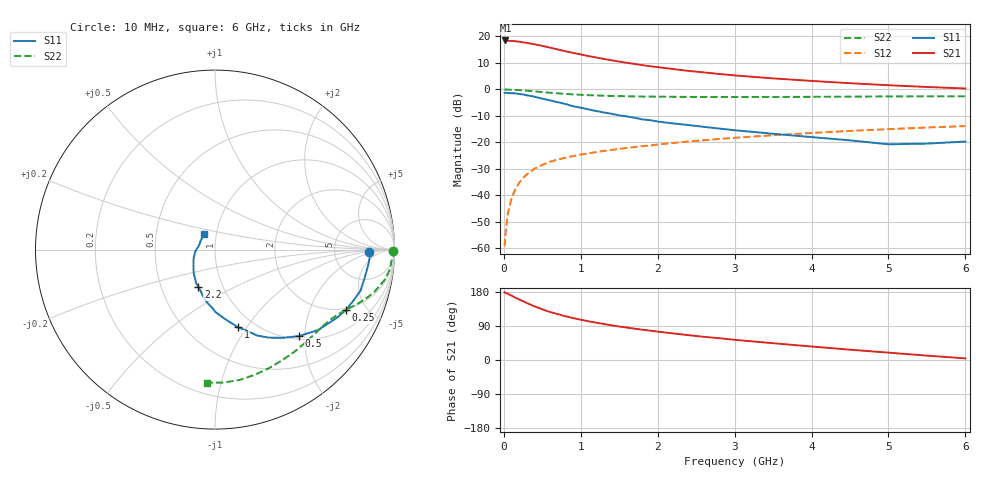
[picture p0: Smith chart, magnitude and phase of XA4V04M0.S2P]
! SIEMENS Discrete & RF Semiconductors
! BFY180
! Si NPN RF Bipolar Junction Transistor in MICRO-X
! VCE = 4 V  IC = 4 mA
! Common Emitter S-Parameters:  May  1997
# GHz  S  MA  R  50
!  f  S11  S21  S12  S22
! GHz  MAG  ANG  MAG  ANG  MAG  ANG  MAG  ANG
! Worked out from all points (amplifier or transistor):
!   36 points, 10 MHz to 6 GHz, reference 50 ohm
!   highest |S21| = 18.5 dB at 20 MHz (marker M1)
!   |S21| within 3 dB of that: start of sweep to 642.7 MHz
!   unconditionally stable (mu >= 1): 1.828 GHz to end of sweep
!   at 250 MHz: K = 0.21, MSG = 25.6 dB, |S12| = -33.4 dB
!   at 1.4 GHz: K = 0.89, MSG = 16.9 dB, |S12| = -22.8 dB
!   at 6 GHz: K = 1.07, MAG = 5.4 dB, |S12| = -13.8 dB
!   S11 on the Smith chart (normalised r, x): 10 MHz: 13, -1; 250 MHz: 1.89, -3.59; 500 MHz: 1.07, -1.87; 1 GHz: 0.84, -0.91; 2.2 GHz: 0.77, -0.34; 6 GHz: 0.87, +0.15
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0.01  0.8582 -0.9  8.31 178.4  0.0011 89.8  0.9896 -0.3
0.02  0.8644 -1.9  8.409 177.4  0.0018 89.6  0.9996 -0.8
0.05  0.8597 -5.0  8.265 174.8  0.0044 86.5  0.9913 -2.1
0.1  0.8488 -10.5  8.255 169.8  0.0089 84.9  0.984 -4.2
0.2  0.8211 -20.4  7.968 159.6  0.0174 79.2  0.9708 -8.1
0.25  0.8029 -24.9  7.744 155.1  0.0213 77.0  0.9603 -10.1
0.3  0.777 -29.4  7.583 150.2  0.025 73.0  0.9463 -11.6
0.4  0.7282 -38.0  7.108 141.5  0.032 69.9  0.9201 -14.7
0.5  0.6719 -45.8  6.645 133.7  0.0377 65.6  0.8916 -17.3
0.6  0.6204 -52.4  6.157 126.6  0.0432 63.4  0.8662 -19.4
0.8  0.5315 -64.1  5.254 115.4  0.0513 58.5  0.8242 -22.9
1  0.4518 -73.5  4.573 106.2  0.0589 56.2  0.7925 -25.8
1.1  0.4202 -77.3  4.268 102.3  0.0622 54.7  0.78 -27.1
1.2  0.3919 -81.6  4.013 98.4  0.0656 54.2  0.7707 -28.4
1.5  0.3239 -92.7  3.362 88.3  0.0754 52.0  0.7478 -32.3
1.7  0.2922 -99.6  3.032 82.6  0.0819 51.2  0.7381 -34.8
2.2  0.2284 -113.9  2.428 70.1  0.0977 48.3  0.7259 -41.5
3  0.1701 -134.4  1.841 53.3  0.1222 43.3  0.7211 -51.9
3.5  0.1455 -146.0  1.617 44.3  0.1365 40.1  0.721 -58.4
4.5  0.1094 -175.7  1.311 27.2  0.1648 32.9  0.7314 -71.9
5.5  0.0949 145.9  1.114 11.5  0.1912 25.1  0.7424 -86.2
6  0.1038 125.4  1.042 4.3  0.2033 20.9  0.7436 -93.5
